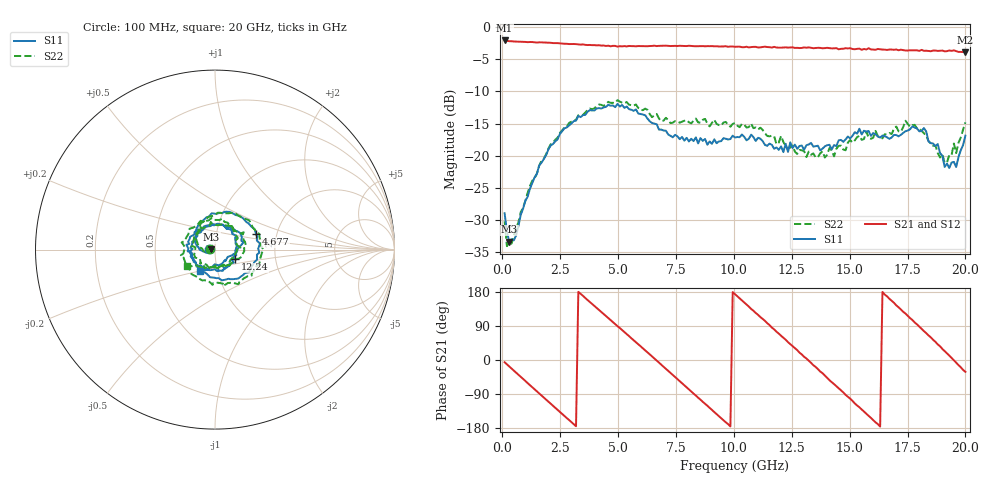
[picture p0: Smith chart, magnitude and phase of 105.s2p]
!Agilent Technologies,N5230C,MY49001569,A.09.33.09
!Agilent N5230C: A.09.33.09
!Date: Wednesday, July 29, 2015 18:53:41
!Correction: S11(Full 2 Port(1,2))
!S21(Full 2 Port(1,2))
!S12(Full 2 Port(1,2))
!S22(Full 2 Port(1,2))
!S2P File: Measurements: S11, S21, S12, S22:
# Hz S  dB  R 50
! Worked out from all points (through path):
!   201 points, 100 MHz to 20 GHz, reference 50 ohm
!   highest |S21| = -2.08 dB at 100 MHz (marker M1); lowest = -3.9 dB at 20 GHz (marker M2)
!   group delay of S21, straight-line fit = 153 ps
!   lowest |S11| = -33.4 dB at 299 MHz (marker M3), VSWR 1.04, Z = 47.9 + j0.0854 ohm
!   |S11| at or under -10 dB: start of sweep to end of sweep
!   |S22| runs from -34.1 to -11.4 dB; largest |S21 - S12| = 0.018
!   S11 on the Smith chart (normalised r, x): 100 MHz: 0.93, +0.01; 4.677 GHz: 1.56, +0.29; 12.24 GHz: 1.24, -0.13; 20 GHz: 0.83, -0.20
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1e8  -28.96 171.3  -2.08 -5.9  -2.06 -6.3  -30.21 171.6
2.99e8  -33.39 177.6  -2.19 -17.1  -2.20 -17.1  -33.45 -179.3
1.095e9  -26.39 -157.6  -2.34 -61.0  -2.32 -60.8  -25.79 -168.3
1.7915e9  -20.53 170.8  -2.40 -99.0  -2.44 -99.0  -20.46 167.0
2.687e9  -15.74 125.6  -2.59 -148.0  -2.58 -147.9  -15.56 117.6
3.483e9  -13.69 81.9  -2.69 169.4  -2.71 169.3  -13.67 77.2
4.677e9  -12.23 20.8  -2.98 105.3  -2.93 105.7  -11.78 16.0
5.473e9  -12.76 -17.8  -2.93 63.1  -2.99 63.0  -12.07 -21.4
6.7665e9  -15.94 -83.3  -2.92 -6.7  -2.94 -6.8  -14.22 -76.9
8.3585e9  -17.15 -177.0  -2.98 -93.8  -2.97 -93.6  -14.22 -152.4
9.254e9  -18.07 130.6  -2.98 -142.6  -2.97 -142.6  -15.05 164.4
1.005e10  -17.17 88.2  -3.07 173.7  -3.08 174.0  -14.94 116.3
1.1244e10  -17.72 30.4  -3.09 108.6  -3.14 107.9  -16.00 51.5
1.2239e10  -18.16 -25.6  -3.15 53.5  -3.19 52.7  -18.47 -7.8
1.3433e10  -18.59 -83.4  -3.28 -13.7  -3.27 -12.7  -19.66 -82.0
1.49255e10  -17.02 -164.4  -3.32 -97.0  -3.29 -97.4  -17.96 170.8
1.5821e10  -16.15 153.0  -3.29 -147.2  -3.49 -147.9  -17.19 121.8
1.67165e10  -17.37 91.5  -3.49 161.6  -3.55 162.0  -16.48 70.5
1.75125e10  -16.09 40.6  -3.65 116.6  -3.58 116.7  -15.08 28.6
1.83085e10  -16.25 11.5  -3.67 70.9  -3.65 71.0  -16.92 -20.5
1.93035e10  -21.92 -45.2  -3.64 11.8  -3.77 11.1  -19.91 -101.8
2e10  -16.89 -125.1  -3.93 -31.3  -3.96 -32.0  -14.82 -150.7
